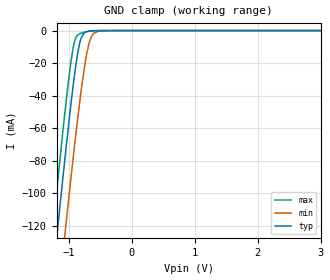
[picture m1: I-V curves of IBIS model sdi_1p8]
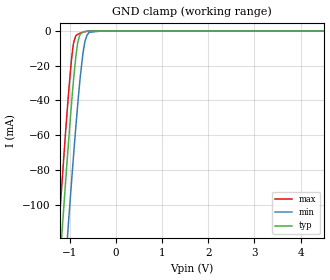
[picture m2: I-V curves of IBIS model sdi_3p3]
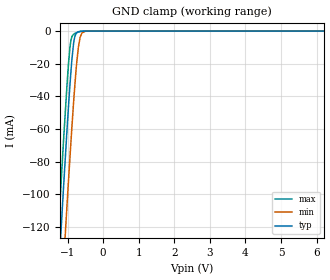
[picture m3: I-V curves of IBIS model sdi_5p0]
|Texas Instruments Incorporated
| Dual, 700kSPS, 16-Bit, Simultaneous Sampling SAR ADC
| Marketing part#   Digital Voltage Range   Package-type   #pins
| ADS8354IPW   1.65V-5.5V   TSSOP   16
| ADS8354IPWR   1.65V-5.5V   TSSOP   16
[IBIS Ver]   4.1
[File name]   ads8354.ibs
[File Rev]   1.1
[Date]   8/8/2016
[Source]
| Texas Instruments Incorporated.
| Analog-eLab Design Center, HPA
| 12500 TI Blvd
| Dallas, TX -75243
[Notes]   Revision History:
| Rev 1.1: 8/8/2016
| - QFN package added.
| Rev 1.0: 12/26/2013
| - Initial version of the model
| - Model generated from simulations in TISPICE
| - Model matched to SPICE simulation
| - C_comp although listed in numerical order of value are
|   obtained from varying PVT conditions. For PVT conditions for
|   each specific value refer the buffer description under
|   respective [Model]. IBIS model user is responsible for using
|   appropriate C_comp to simulate for Signal Integrity.
[Disclaimer]
| This model is designed as an aid for customers of Texas Instruments.
| TI and its licensors and suppliers make no warranties, either expressed
| or implied, with respect to this  model, including the warranties of
| merchantability or fitness for a particular purpose. The model is
| provided solely on an "as is" basis. The entire risk as to its quality
| and performance is with the customer.
[Copyright]
(C) Copyright 2013 Texas Instruments Incorporated.All rights reserved.
|   ADS8354
[Component]   ADS8354PW
[Manufacturer]   TI
[Package]   |16 TSSOP  -  PW package
|   typ   min   max
R_pkg   0.14389   0.13702   0.16381
L_pkg   1.96144nH   1.83315nH   2.40982nH
C_pkg   0.37623pF   0.34690pF   0.47625pF
[Pin]  signal_name   model_name   R_pin   L_pin   C_pin
1   AINP_A   NC   0.14441   2.71929nH  0.46906pF
2   AINM_A   NC   0.15355   2.32903nH  0.47433pF
3   REFIO_A   NC   0.13911   1.85326nH  0.34789pF
4   REFGND_A   NC   0.14415   1.88929nH  0.35653pF
5   REFGND_B   NC   0.14337   1.88150nH  0.35622pF
6   REFIO_B   NC   0.13903   1.85256nH  0.34801pF
7   AINM-B   NC   0.15963   2.37622nH  0.47576pF
8   AINP_B   NC   0.15200   2.78385nH  0.47248pF
9   DVDD   POWER   0.14727   2.74603nH  0.47071pF
10   SDI   SDI   0.16381   2.40982nH  0.47625pF
11   _CS   SDI   0.14405   1.89362nH  0.34932pF
12   SCLK   SDI   0.13724   1.83315nH  0.35457pF
13   SDO_A   SDO   0.13731   1.83428nH  0.35410pF
14   SDO_B   SDO   0.13702   1.83634nH  0.34690pF
15   GND   GND   0.08558   2.05285nH  0.50745pF
16   AVDD   POWER   0.08145   2.44314nH  0.49737pF
[Component]   ADS8354RTE
[Manufacturer]   TI
[Package]  |16 QFN   RTE package
|   typ   min   max
R_pkg   0.067   0.027   0.083
L_pkg   0.937nH   0.593nH   1.143nH
C_pkg   0.144pF   0.126pF   0.200pF
[Pin]  signal_name   model_name   R_pin   L_pin   C_pin
1   REFIO_A   NC   NA   NA   NA
2   REFGND_A   NC   NA   NA   NA
3   REFGND_B   NC   NA   NA   NA
4   REFIO_B   NC   NA   NA   NA
5   AINM_B   NC   NA   NA   NA
6   AINP_B   NC   NA   NA   NA
7   DVDD   POWER   NA   NA   NA
8   SDI   SDI   NA   NA   NA
9   _CS   SDI   NA   NA   NA
10   SCLK   SDI   NA   NA   NA
11   SDO_A   SDO   NA   NA   NA
12   SDO_B   SDO   NA   NA   NA
13   GND   GND   NA   NA   NA
14   AVDD   POWER   NA   NA   NA
15   AINP_A   NC   NA   NA   NA
16   AINM_A   NC   NA   NA   NA
|   Model Selectors
[Model Selector] SDI
sdi_1p8   1.8V  digital input
sdi_3p3   3.3V  digital input
sdi_5p0   5.0V  digital input
[Model Selector] SDO
sdo_1p8   1.8V  digital tristate
sdo_3p3   3.3V  digital tristate
sdo_5p0   5.0V  digital tristate
| Models and submodels in the file (6): sdi_1p8 (Input), sdi_3p3 (Input), sdi_5p0 (Input), sdo_1p8 (3-state), sdo_3p3 (3-state), sdo_5p0 (3-state)
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|   sdi_1p8 Model
[Model]   sdi_1p8
Model_type   Input
Vinl = 0.54
Vinh = 1.26
|   typ   min   max
|   (nom PVT)   (fast PVT)   (slow PVT)
C_comp   3.893e-13   3.165e-13   4.681e-13
[Model spec]
|subparameter
Vinl   0.54   0.495   0.585
Vinh   1.26   1.155   1.365
| Where nom  PVT is Nominal Process, 1.8V, 27C
|   Fast PVT is Strong Process,  1.95V, -40C
|   Slow PVT is Weak Process,   1.65V, 125C
[Voltage Range]   1.8   1.65   1.95
|Junction Temperature
[Temperature Range]   27   125   -40
[Power Clamp Reference]   1.8   1.65   1.95
[GND Clamp Reference]   0   0   0
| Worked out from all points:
|   GND clamp passes 1 mA (typ) near -0.74 V on its own axis
[GND Clamp]
|   Voltage   I(typ)   I(min)   I(max)
-1.8V     -365.8mA   -409.6mA   -339.5mA
-1.389V   -202mA     -248mA     -174mA
-1.18V    -121mA     -167.7mA   -92.21mA
-1.091V   -87.51mA   -134.2mA   -58.87mA
-1.046V   -71.26mA   -117.8mA   -43.03mA
-937.1mV  -34.31mA   -78.89mA   -10.91mA
-833.4mV  -8.006mA   -44.56mA   -1.995mA
-755.6mV  -1.288mA   -22.45mA   -1.045mA
-682.6mV  -321.2uA   -7.802mA   -460.3uA
-610.5mV  -81.74uA   -1.624mA   -133.9uA
-513mV    -8.174uA   -152.9uA   -11.17uA
3.6V      0A         0A         0A
[POWER Clamp]
|   Voltage   I(typ)   I(min)   I(max)
-1.8V     0A         0A         0A
-306.8mV  0A         0A         0A
3.6V      0A         0A         0A
|   sdi_3p3 Model
[Model]   sdi_3p3
Model_type   Input
Vinl = 0.99
Vinh = 2.31
|   typ   min   max
|   (nom PVT)   (fast PVT)   (slow PVT)
C_comp   3.637e-13   3.022e-13   4.321e-13
[Model spec]
|subparameter
Vinl   0.99   0.9   1.08
Vinh   2.31   2.1   2.52
| Where nom  PVT is Nominal Process, 3.3V, 27C
|   Fast PVT is Strong Process,  3.6V, -40C
|   Slow PVT is Weak Process,   3V, 125C
[Voltage Range]   3.3   3   3.6
|Junction Temperature
[Temperature Range]   27   125   -40
[Power Clamp Reference]   3.3   3   3.6
[GND Clamp Reference]   0   0   0
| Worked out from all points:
|   GND clamp passes 1 mA (typ) near -0.74 V on its own axis
[GND Clamp]
|   Voltage   I(typ)   I(min)   I(max)
-3.3V     -977.1mA   -1.014A    -955.8mA
-1.611V   -290mA     -334.8mA   -262.9mA
-1.219V   -136mA     -182.6mA   -107.3mA
-1.209V   -132.1mA   -178.7mA   -103.3mA
-1.097V   -89.83mA   -136.6mA   -61.16mA
-1.044V   -70.62mA   -117.1mA   -42.41mA
-915mV    -27.6mA    -71.3mA    -6.969mA
-834mV    -8.108mA   -44.75mA   -2.005mA
-788.7mV  -2.831mA   -31.29mA   -1.387mA
-686.4mV  -342.9uA   -8.352mA   -484.4uA
-576mV    -38.3uA    -701.8uA   -61.61uA
6.6V      0A         0A         0A
[POWER Clamp]
|   Voltage   I(typ)   I(min)   I(max)
-3.3V     0A         0A         0A
-3.03V    0A         0A         0A
6.6V      0A         0A         0A
|   sdi_5p0 Model
[Model]   sdi_5p0
Model_type   Input
Vinl = 1.5
Vinh = 3.5
|   typ   min   max
|   (nom PVT)   (fast PVT)   (slow PVT)
C_comp   3.444e-13   2.913e-13   4.063e-13
[Model spec]
|subparameter
Vinl   1.5   1.35   1.65
Vinh   3.5   3.15   3.85
| Where nom  PVT is Nominal Process, 5V, 27C
|   Fast PVT is Strong Process,  5.5V, -40C
|   Slow PVT is Weak Process,   4.5V, 125C
[Voltage Range]   5   4.5   5.5
|Junction Temperature
[Temperature Range]   27   125   -40
[Power Clamp Reference]   5   4.5   5.5
[GND Clamp Reference]   0   0   0
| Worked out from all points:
|   GND clamp passes 1 mA (typ) near -0.74 V on its own axis
[GND Clamp]
|   Voltage   I(typ)   I(min)   I(max)
-5V       -1.676A    -1.707A    -1.659A
-1.26V    -151.7mA   -198.2mA   -123.1mA
-1.2V     -128.4mA   -175.1mA   -99.7mA
-1.107V   -93.79mA   -140.5mA   -65.08mA
-1.015V   -60.34mA   -106.6mA   -32.68mA
-932mV    -32.74mA   -77.14mA   -9.894mA
-875mV    -16.69mA   -57.88mA   -3.225mA
-825.5mV  -6.768mA   -42.13mA   -1.864mA
-698mV    -420.6uA   -10.2mA    -563.7uA
-594.5mV  -58.01uA   -1.102mA   -94.85uA
-455mV    -1.715uA   -35.38uA   -1.789uA
10V       0A         0A         0A
[POWER Clamp]
|   Voltage   I(typ)   I(min)   I(max)
-5V       0A         0A         0A
-4.83V    0A         0A         0A
10V       0A         0A         0A
